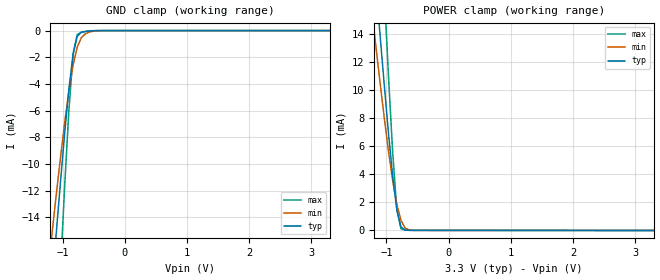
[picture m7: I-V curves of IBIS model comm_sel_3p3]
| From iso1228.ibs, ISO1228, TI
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|   Model comm_sel_3p3
[Model] comm_sel_3p3
Model_type Input
Vinl =  0.990V
Vinh =  2.310V
C_comp   0.525pF   0.628pF   0.413pF
[Model Spec]
Vinh   2.310V   2.100V   2.520V
Vinl   0.990V   0.900V   1.080V
[Temperature Range]   27.000   0.150k   -40.000
[Voltage Range]   3.300V   3.000V   3.600V
[POWER Clamp Reference]   3.300V   3.000V   3.600V
[GND Clamp Reference]   0.0V   0.0V   0.0V
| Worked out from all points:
|   GND clamp passes 1 mA (typ) near -0.79 V on its own axis
|   POWER clamp passes 1 mA (typ) near -0.81 V on its own axis
[GND_clamp]
|Voltage   I(typ)   I(min)   I(max)
-3.3V     -218.7mA   -148.2mA   -389.8mA
-1.167V   -18.85mA   -15mA      -30.74mA
-1.1V     -14.96mA   -12.15mA   -24.14mA
-1.033V   -11.2mA    -9.409mA   -17.7mA
-967mV    -7.614mA   -6.833mA   -11.53mA
-900mV    -4.363mA   -4.512mA   -5.943mA
-833mV    -1.786mA   -2.578mA   -1.74mA
-767mV    -434.7uA   -1.254mA   -297uA
-700mV    -119.6uA   -524.2uA   -125.9uA
-567mV    -22.22uA   -106.1uA   -33.31uA
-367mV    -808.9nA   -5.984uA   -992.2nA
3.3V      0A         0A         0A
[POWER_clamp]
|Voltage   I(typ)   I(min)   I(max)
-3.3V     208mA      137.3mA    378.9mA
-1.233V   21.08mA    15.67mA    35.84mA
-1.167V   17.4mA     13.03mA    29.42mA
-1.1V     13.79mA    10.45mA    23.09mA
-1.033V   10.27mA    7.968mA    16.91mA
-967mV    6.922mA    5.635mA    10.98mA
-900mV    3.876mA    3.548mA    5.562mA
-833mV    1.47mA     1.861mA    1.484mA
-767mV    257.1uA    723.6uA    126.2uA
-700mV    30.79uA    176.7uA    18.56uA
-567mV    8.014uA    10.43uA    10.82uA
3.3V      0A         0A         776nA
